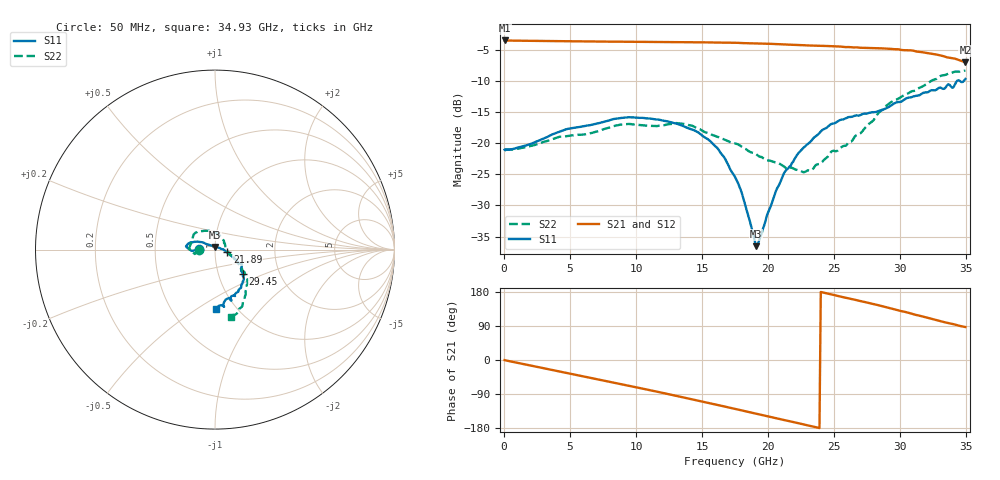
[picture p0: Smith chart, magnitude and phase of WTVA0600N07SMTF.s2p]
! 50 ohm 2-Port S-parameters measured by Modelithics Inc support@modelithics.com  Tampa, FL USA 813-866-6335 (February 2024)
! Smiths Interconnect,  6dB P/N: WTVA0600N07SMTF, Temperature: 125 C
! Board: 10 mil Rogers 4350B, Mounting Pad Dimensions: Length: 15 mils, Width: 25 mils, Gap: 40 mils.
# Hz S RI R 50
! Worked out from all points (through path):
!   352 points, 50 MHz to 34.93 GHz, reference 50 ohm
!   highest |S21| = -3.41 dB at 100 MHz (marker M1); lowest = -6.9 dB at 34.93 GHz (marker M2)
!   group delay of S21, straight-line fit = 21.6 ps
!   lowest |S11| = -36.6 dB at 19.11 GHz (marker M3), VSWR 1.03, Z = 50.1 + j1.48 ohm
!   |S11| at or under -10 dB: start of sweep to 34.27 GHz; 34.55 GHz to 34.77 GHz (223.7 MHz wide, 0.645 % of centre)
!   |S22| runs from -24.6 to -8.2 dB; largest |S21 - S12| = 0.0076
!   S11 on the Smith chart (normalised r, x): 50 MHz: 0.84, +0.00; 21.89 GHz: 1.15, -0.04; 29.45 GHz: 1.30, -0.38; 34.93 GHz: 0.81, -0.60
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5e7  -0.0889 0.000859  0.6754 -0.00434  0.6743 -0.00419  -0.0873 -0.00104
1e8  -0.0895 0.000177  0.6754 -0.00916  0.6744 -0.00921  -0.0885 -0.000745
2.787e9  -0.107 -0.00234  0.6286 -0.2306  0.6274 -0.2306  -0.1001 -0.012
5.8715e9  -0.1366 -0.00241  0.4923 -0.4467  0.4915 -0.4462  -0.1155 -0.0214
8.956e9  -0.1599 0.0152  0.2848 -0.5949  0.2836 -0.5942  -0.1424 0.00208
1.1742e10  -0.1523 0.03  0.0595 -0.654  0.058 -0.6531  -0.1278 0.0546
1.3533e10  -0.1322 0.0414  -0.0952 -0.6488  -0.0966 -0.6477  -0.1098 0.0934
1.54235e10  -0.0987 0.0447  -0.2538 -0.6007  -0.256 -0.5984  -0.062 0.1045
1.66175e10  -0.0678 0.0399  -0.3447 -0.5494  -0.3455 -0.548  -0.0289 0.1042
1.7513e10  -0.0443 0.0292  -0.4088 -0.5015  -0.4087 -0.5002  -0.0086 0.0995
1.80105e10  -0.0299 0.0259  -0.4414 -0.4686  -0.4404 -0.4679  0.00355 0.0936
1.9105e10  0.00165 0.0148  -0.5016 -0.3956  -0.501 -0.3949  0.0284 0.0767
2.05975e10  0.0416 0.0028  -0.5658 -0.2805  -0.5653 -0.2794  0.0476 0.0518
2.11945e10  0.0571 -0.00665  -0.5829 -0.231  -0.5821 -0.2302  0.0509 0.0407
2.1891e10  0.0695 -0.0153  -0.5978 -0.1753  -0.5973 -0.174  0.055 0.0305
2.33835e10  0.1001 -0.0431  -0.6131 -0.0471  -0.6122 -0.0472  0.0623 -0.000378
2.5473e10  0.1357 -0.0745  -0.5881 0.1324  -0.5871 0.1323  0.0869 -0.0311
2.91545e10  0.1522 -0.1252  -0.4259 0.3921  -0.4213 0.3954  0.1656 -0.1285
2.9453e10  0.1546 -0.1378  -0.4049 0.4094  -0.3993 0.4135  0.1674 -0.1432
3.25375e10  0.1256 -0.2367  -0.155 0.5014  -0.1513 0.5015  0.1605 -0.284
3.39305e10  0.0748 -0.2705  -0.0447 0.484  -0.0409 0.4836  0.1277 -0.3505
3.49255e10  0.00767 -0.3306  0.0234 0.45  0.0238 0.449  0.0893 -0.3765
